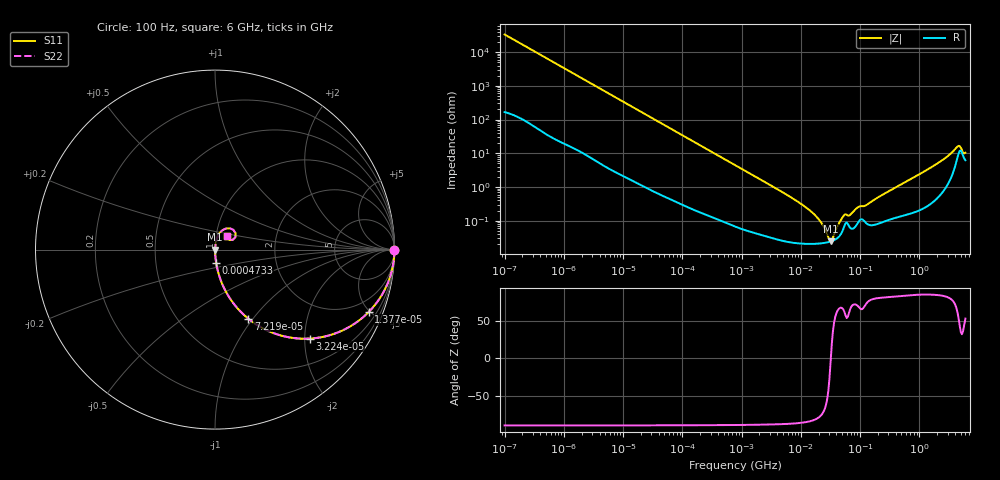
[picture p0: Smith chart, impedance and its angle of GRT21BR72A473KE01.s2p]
!Murata Part Number: GRT21BR72A473KE01
!These Parameters are Measured in Series Mode Connection
!Data Generated on Jun 19, 2026
!  o--ll--o
!Port1  Port2
!  o------o
!Operation Temp=25[degC], DC Bias Voltage=0[V]
!Freq. Start=100[Hz] Stop=6[GHz] 401[Steps]
# Hz S RI R 50
!Freq.(Hz) S11(Real) S11(Imag) S21(Real) S21(Imag) S12(Real) S12(Imag) S22(Real) S22(Imag)
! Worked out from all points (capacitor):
!   401 points, 100 Hz to 6 GHz, reference 50 ohm
!   read as one part in series: C = 47.7 nF near 109 Hz
!   lowest |Z| = 24.3 mohm at 31.85 MHz (marker M1)
!   series resonance near 32.11 MHz, so ESL is about 510 pH
!   S11 on the Smith chart (normalised r, x): 100 Hz: open; 13.77 kHz: 1.03, -4.93; 32.24 kHz: 1.01, -2.11; 72.19 kHz: 1.01, -0.95; 473.3 kHz: 1.00, -0.15; 6 GHz: 1.12, +0.17
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100  1 -0.003  2.4e-05 0.003  2.4e-05 0.003  1 -0.003
2008  0.9961 -0.0593  0.00391 0.0593  0.00391 0.0593  0.9961 -0.0593
6728  0.9609 -0.1908  0.0391 0.1908  0.0391 0.1908  0.9609 -0.1908
13772  0.857 -0.3468  0.143 0.3468  0.143 0.3468  0.857 -0.3468
32244  0.5271 -0.4957  0.4729 0.4957  0.4729 0.4957  0.5271 -0.4957
40335  0.4173 -0.4895  0.5827 0.4895  0.5827 0.4895  0.4173 -0.4895
72189  0.1851 -0.3843  0.8149 0.3843  0.8149 0.3843  0.1851 -0.3843
147774  0.053 -0.2193  0.947 0.2193  0.947 0.2193  0.053 -0.2193
473344  0.00624 -0.0725  0.9938 0.0725  0.9938 0.0725  0.00624 -0.0725
774597  0.00267 -0.0446  0.9973 0.0446  0.9973 0.0446  0.00267 -0.0446
6644369  0.000255 -0.00509  0.9997 0.00509  0.9997 0.00509  0.000255 -0.00509
1.555665e7  0.000209 -0.00175  0.9998 0.00175  0.9998 0.00175  0.000209 -0.00175
2.225763e7  0.000215 -0.000838  0.9998 0.000838  0.9998 0.000838  0.000215 -0.000838
3.184506e7  0.000243 -1.87e-05  0.9998 1.87e-05  0.9998 1.87e-05  0.000243 -1.87e-05
5.449875e7  0.000705 0.00132  0.9993 -0.00132  0.9993 -0.00132  0.000705 0.00132
6.817316e7  0.000616 0.00137  0.9994 -0.00137  0.9994 -0.00137  0.000616 0.00137
9.326766e7  0.000902 0.00239  0.9991 -0.00239  0.9991 -0.00239  0.000902 0.00239
1.275994e8  0.000851 0.00279  0.9991 -0.00279  0.9991 -0.00279  0.000851 0.00279
3.124326e8  0.00113 0.00757  0.9989 -0.00757  0.9989 -0.00757  0.00113 0.00757
1.873145e9  0.00618 0.0453  0.9938 -0.0453  0.9938 -0.0453  0.00618 0.0453
4.385646e9  0.0829 0.1186  0.9171 -0.1186  0.9171 -0.1186  0.0829 0.1186
6e9  0.0644 0.0731  0.9356 -0.0731  0.9356 -0.0731  0.0644 0.0731
